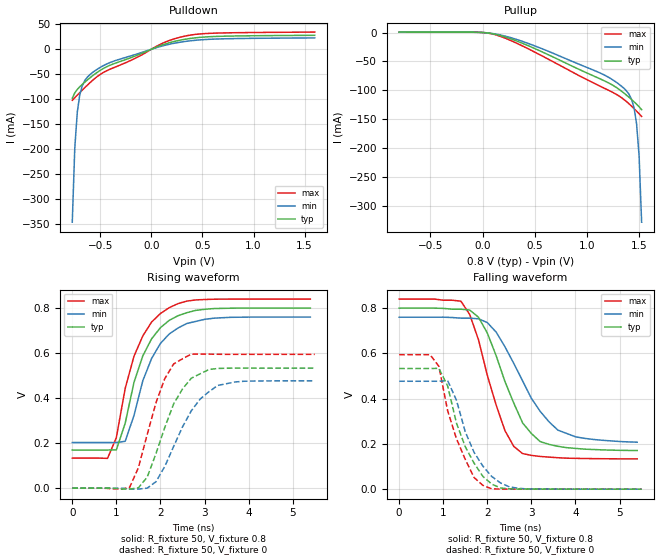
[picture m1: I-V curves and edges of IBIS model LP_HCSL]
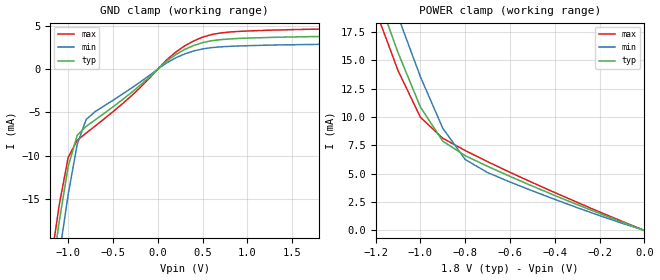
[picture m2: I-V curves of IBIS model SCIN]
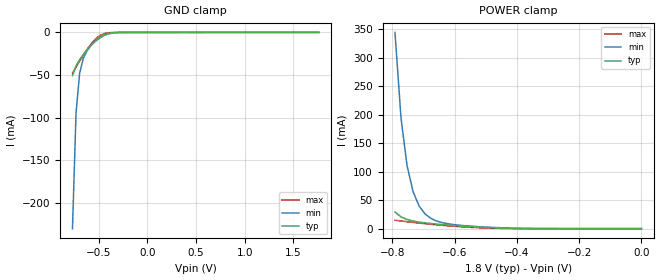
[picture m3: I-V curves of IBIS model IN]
| Integrated Devices Technolgy, Inc
[IBIS Ver]   4.1
[File name]   9dbu0431.ibs
[File Rev]   1.0
[Date]   Oct. 09, 2014
[Disclaimer] Integrated Device Technology, Inc. ("IDT") hereby grants the
   user of this ibis model a non-exclusive, nontransferable
   license to use this ibis model under the following terms. the
   user is granted this license only to use the ibis model and is
   not granted rights to sell, copy (except as needed to run the
   ibis model), rent, lease or sub-license the ibis model in
   whole or in part, or in modified form to anyone. the user may
   modify the ibis model to suit its specific applications, but
   rights to derivative works and such modifications shall belong
   to idt. this ibis model is provided on an as is" basis and idt
   makes absolutely no warranty with respect to the information
   contained herein. idt disclaims and customer waives all
   warranties, express and implied, including warranties of
   merchantability and fitness for a particular purpose. the
   entire risk as to quality and performance is with the user
   accordingly, in no event shall idt be liable for any direct or
   indirect damages, whether in contract or tort, including any
   lost profits or other incidental, consequential, exemplary, or
   punitive damages arising out of the use or application of the
   ibis model. further, idt reserves the right to make changes
   without notice to any product herein to improve reliability,
   function, or design. idt does not convey any license under
   patent rights or any other intellectual property rights,
   including those of third parties. idt is not obligated to
   provide maintenance or support for the licensed ibis model.
[Copyright]   Copyright 2012, Integrated Devices Technolgy, Inc. all rights
   reserved
[Component]   9dbu0431
[Manufacturer] Integrated Device Technology, Inc.
[Package]
|32-VFQFPN
|variable   typ   min   max
R_pkg   81.1m   62.2m   100.0m
L_pkg   6.7nH   4.9nH   8.5nH
C_pkg   0.53pF   0.21pF   0.85pF
[Pin] signal_name  model_name
1 ^vHIBW_BYPM_LOBW#   IN
2 FB_DNC   LP_HCSL
3 FB_DNC#   LP_HCSL
4 VDDR1.5   POWER
5 CLK_IN   CLKIN
6 CLK_IN#   CLKIN
7 GNDR   GND
8 GNDDIG   GND
9 VDDDIG1.5   POWER
10 SCLK_3.3   SCIN
11 SDATA_3.3   SCIN
12 vOE0#   IN
13 DIF0   LP_HCSL
14 DIF0#   LP_HCSL
15 GND   GND
16 VDDO1.5   POWER
17 vOE1#   IN
18 DIF1   LP_HCSL
19 DIF1#   LP_HCSL
20 GNDA   GND
21 VDDA1.5   POWER
22 DIF2   LP_HCSL
23 DIF2#   LP_HCSL
24 vOE2#   IN
25 VDDO1.5   POWER
26 GND   GND
27 DIF3   LP_HCSL
28 DIF3#   LP_HCSL
29 vOE3#   IN
30 GND   GND
31 ^CKPWRGD_PD#   PD
32 SADR_tri   IN
[Diff Pin]  inv_pin  vdiff tdelay_typ tdelay_min  tdelay_max
13   14   NA   0   0   0
17   18   NA   0   0   0
| Models and submodels in the file (5): LP_HCSL (Output), SCIN (Input), IN (Input), CLKIN (Input), PD (Input)
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[Model]   LP_HCSL
Model_type   Output
Polarity   Non-Inverting
|   typ   min   max
C_comp   2pF   1.5pF   2.5pF
Vmeas = 0.4V
Rref = 50
Cref = 0
Vref = 0.4V
|   typ   min   max
[Voltage range]   0.8V   0.76V   0.84V
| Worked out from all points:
|   slope of the pulldown table from 0 to 0.12 V, typ, clamps not added: 12.6 ohm
|   slope of the pullup table from 0 to 0.12 V, typ, clamps not added: 40.4 ohm
|   rising waveform, R_fixture 50, V_fixture 0.8: 20-80 % time 633ps typ, 641ps min, 627ps max; typ from 0.169 V to 0.8 V
|   falling waveform, R_fixture 50, V_fixture 0.8: 20-80 % time 760ps typ, 973ps min, 640ps max; typ from 0.8 V to 0.171 V
|   rising waveform, R_fixture 50, V_fixture 0: 20-80 % time 648ps typ, 750ps min, 540ps max; typ from 0 V to 0.533 V
|   falling waveform, R_fixture 50, V_fixture 0: 20-80 % time 591ps typ, 611ps min, 563ps max; typ from 0.533 V to 0 V
[Pulldown]
|Voltage   I (typ)   I (min)   I (max)
|Note, modeling breaks down at 250mA and above.  This is well beyond the functional   |
|operating range of the device.  Should this scenario occur, catastrophic failure and   |
|possible damage to the device and/or board is of higher concern than the I-V curve   |
|behavior.  The IBIS checker will flag currents in excess of 10A with warnings.  Lines   |
|with currents in excess of 0.35 A have been commented out.  The points still remain|
|available to the user if the user desires to use them.   |
|-8.00000e-01   -1.18956e-01   -6.48321e-01   -1.07624e-01
-775.5mV  -98.23mA   -346.4mA   -102.3mA
-751mV    -87.43mA   -198mA     -97.14mA
-726.5mV  -80.52mA   -126.3mA   -92.02mA
-702mV    -75.15mA   -91.19mA   -86.94mA
-677.6mV  -70.41mA   -73.06mA   -81.92mA
-628.6mV  -61.7mA    -56.11mA   -72.13mA
-579.6mV  -53.61mA   -47.04mA   -62.91mA
-359.2mV  -28.39mA   -23.18mA   -36.07mA
106.1mV   8.578mA    6.556mA    11.68mA
326.5mV   19.84mA    15.45mA    26.21mA
620.4mV   25.5mA     20.31mA    32.18mA
1.6V      27.87mA    22.65mA    34.32mA
[Pullup]
|Voltage   I (typ)   I (min)   I (max)
|Note, modeling breaks down at 250mA and above.  This is well beyond the functional   |
|operating range of the device.  Should this scenario occur, catastrophic failure and   |
|possible damage to the device and/or board is of higher concern than the I-V curve   |
|behavior.  The IBIS checker will flag currents in excess of 10A with warnings.  Lines   |
|with currents in excess of 0.35 A have been commented out.  The points still remain|
|available to the user if the user desires to use them.   |
-800mV    720.8uA    674uA      687.8uA
-48.48mV  366.7uA    329uA      361.2uA
121.2mV   -3.014mA   -2.451mA   -3.786mA
606.1mV   -36.3mA    -30.55mA   -43.69mA
1.139V    -80.99mA   -70.87mA   -93.7mA
1.309V    -98.03mA   -89.24mA   -109.6mA
1.406V    -112mA     -106.7mA   -123.2mA
1.43V     -115.8mA   -115.3mA   -127.2mA
1.455V    -119.8mA   -130mA     -131.5mA
1.479V    -123.9mA   -157.7mA   -135.9mA
1.503V    -128.3mA   -213.4mA   -140.4mA
1.527V    -133.4mA   -327.8mA   -145mA
| 1.55152e+00   -1.40006e-01   -5.61449e-01   -1.49713e-01
| 1.57576e+00   -1.50454e-01   -1.02014e+00   -1.54462e-01
| 1.60000e+00   -1.70613e-01   -1.84947e+00   -1.59268e-01
[Ramp]
|   typ   min   max
dV/dt_r   0.322/0.652n   0.288/0.756n   0.359/0.544n
dV/dt_f   0.377/0.759n   0.331/0.973n   0.423/0.64n
R_load =   50
[Rising Waveform]
R_fixture = 50
V_fixture = 0.8   |Vcc_typ
V_fixture_min = 0.76 |Vcc_min
V_fixture_max = 0.84 |Vcc_max
C_fixture = 0.0p
| Time   typ   min   max
0s        169.4mV    202.7mV    133.6mV
800ps     169.4mV    202.7mV    132.5mV
1ns       170.3mV    202.6mV    224.9mV
1.2ns     288.2mV    208.4mV    442.8mV
1.4ns     470.3mV    322.9mV    586.2mV
1.6ns     587.8mV    477.4mV    676.4mV
2ns       713mV      643mV      775.9mV
2.4ns     766.1mV    711.6mV    819.8mV
3ns       794.4mV    749.8mV    837.9mV
5.4ns     800mV      760mV      840mV
[Falling Waveform]
R_fixture = 50
V_fixture = 0.8   |Vcc_typ
V_fixture_min = 0.76 |Vcc_min
V_fixture_max = 0.84 |Vcc_max
C_fixture = 0.0p
| Time   typ   min   max
0s        800mV      760mV      840mV
1.4ns     795.4mV    755.9mV    830.8mV
1.6ns     791.6mV    755.7mV    772.3mV
1.8ns     759.8mV    753mV      660mV
2ns       689.9mV    736.2mV    503mV
2.4ns     475.8mV    629.3mV    258.6mV
2.8ns     292.8mV    478.6mV    157.3mV
3.2ns     210.1mV    343.6mV    144.6mV
3.6ns     189.4mV    261mV      139mV
5.4ns     170.7mV    207.6mV    133.8mV
[Rising Waveform]
R_fixture = 50
V_fixture = 0
C_fixture = 0.0p
| Time   typ   min   max
0s        36.65nV    422.2nV    16.59nV
1.3ns     -4.214mV   -3.249mV   3.128mV
1.5ns     1.766mV    -4.053mV   90.98mV
1.7ns     49.12mV    109.5uV    238.7mV
1.9ns     154.6mV    29.05mV    380.5mV
2.1ns     270.8mV    97.03mV    487.3mV
2.5ns     440.5mV    272.2mV    574.7mV
2.9ns     507.8mV    395.6mV    595.4mV
3.3ns     531.7mV    456.3mV    594.8mV
5.5ns     533mV      476.8mV    594.4mV
[Falling Waveform]
R_fixture = 50
V_fixture = 0
C_fixture = 0.0p
| Time   typ   min   max
0s        533mV      476.9mV    594.4mV
700ps     533mV      476.9mV    594.2mV
900ps     534.1mV    476.8mV    543.6mV
1.1ns     456.1mV    479.9mV    346.4mV
1.3ns     292mV      393mV      223.1mV
1.5ns     187.5mV    253.1mV    131.6mV
1.9ns     56.28mV    101.6mV    16.79mV
2.3ns     5.253mV    27.26mV    387.4uV
2.7ns     410.2uV    4.104mV    300.6uV
5.5ns     22.66uV    49.02uV    7.861uV
|   Model SCIN
[Model]   SCIN
Model_type   Input
Vinl =   0.54V
Vinh =   1.26V
C_comp   3.40pF   2.85pF   3.95pF
[Temperature Range]   25.00   70.00   0.000
[Voltage Range]   1.80V   1.62V   1.98V
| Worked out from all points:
|   GND clamp passes 1 mA (typ) near -0.10 V on its own axis
|   POWER clamp passes 1 mA (typ) near -0.13 V on its own axis
[GND_clamp]
| voltage   I(typ)   I(min)   I(max)
-1.8V     -72.89mA   -76.87mA   -70.76mA
-1.2V     -24.92mA   -29.01mA   -22.79mA
-1.1V     -17.6mA    -21.48mA   -15.68mA
-1V       -11.25mA   -14.47mA   -10.2mA
-900mV    -7.66mA    -8.72mA    -8.23mA
-800mV    -6.62mA    -5.82mA    -7.39mA
-300mV    -2.76mA    -2.24mA    -3.14mA
100mV     920uA      720uA      1.08mA
300mV     2.27mA     1.75mA     2.68mA
600mV     3.28mA     2.48mA     3.99mA
900mV     3.54mA     2.67mA     4.35mA
1.8V      3.76mA     2.86mA     4.62mA
[POWER_clamp]
| voltage   I(typ)   I(min)   I(max)
-1.8V     57.31mA    60.73mA    55.47mA
-1.2V     21.16mA    24.54mA    19.4mA
-1.1V     15.67mA    18.87mA    14.09mA
-1V       10.87mA    13.54mA    9.97mA
-900mV    7.86mA     9mA        8.12mA
-800mV    6.59mA     6.25mA     7.04mA
-700mV    5.65mA     5.1mA      6.06mA
-600mV    4.76mA     4.27mA     5.12mA
-300mV    2.28mA     2.01mA     2.48mA
0V        44.83pA    370pA      23.45pA
|   Model IN
[Model]   IN
Model_type   Input
Polarity   Non-Inverting
Vinl = 0.63V
Vinh = 1.17V
|   typ   min   max
C_comp   2pF   1.5pF   2.5pF
|   typ   min   max
[Voltage range]   1.8V   1.7V   1.9V
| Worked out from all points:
|   GND clamp passes 1 mA (typ) near -0.39 V on its own axis
|   POWER clamp passes 1 mA (typ) near -0.45 V on its own axis
[GND_clamp]
|Voltage   I (typ)   I (min)   I (max)
|Note, modeling breaks down at 250mA and above.  This is well beyond the functional   |
|operating range of the device.  Should this scenario occur, catastrophic failure and   |
|possible damage to the device and/or board is of higher concern than the I-V curve   |
|behavior.  The IBIS checker will flag currents in excess of 10A with warnings.  Lines   |
|with currents in excess of 0.35 A have been commented out.  The points still remain|
|available to the user if the user desires to use them.   |
|-1.80000e+00   -4.43726e+01   -4.17458e+01   -4.86820e+01
|-1.76327e+00   -4.25922e+01   -4.02056e+01   -4.65395e+01
|-1.72653e+00   -4.08117e+01   -3.86654e+01   -4.43969e+01
|-1.68980e+00   -3.90312e+01   -3.71251e+01   -4.22544e+01
|-1.65306e+00   -3.72507e+01   -3.55849e+01   -4.01118e+01
|-1.61633e+00   -3.54702e+01   -3.40446e+01   -3.79693e+01
|-1.57959e+00   -3.36896e+01   -3.25043e+01   -3.58267e+01
|-1.54286e+00   -3.19091e+01   -3.09640e+01   -3.36840e+01
|-1.50612e+00   -3.01285e+01   -2.94236e+01   -3.15414e+01
|-1.46939e+00   -2.83479e+01   -2.78833e+01   -2.93987e+01
|-1.43265e+00   -2.65672e+01   -2.63429e+01   -2.72561e+01
|-1.39592e+00   -2.47866e+01   -2.48025e+01   -2.51134e+01
|-1.35918e+00   -2.30059e+01   -2.32621e+01   -2.29707e+01
|-1.32245e+00   -2.12253e+01   -2.17217e+01   -2.08279e+01
|-1.28571e+00   -1.94446e+01   -2.01813e+01   -1.86852e+01
|-1.24898e+00   -1.76639e+01   -1.86409e+01   -1.65424e+01
|-1.21224e+00   -1.58832e+01   -1.71005e+01   -1.43996e+01
|-1.17551e+00   -1.41025e+01   -1.55600e+01   -1.22568e+01
|-1.13878e+00   -1.23218e+01   -1.40196e+01   -1.01141e+01
|-1.10204e+00   -1.05411e+01   -1.24792e+01   -7.97124e+00
|-1.06531e+00   -8.76046e+00   -1.09388e+01   -5.82843e+00
|-1.02857e+00   -6.97978e+00   -9.39848e+00   -3.68562e+00
|-9.91837e-01   -5.19912e+00   -7.85813e+00   -1.54785e+00
|-9.55102e-01   -3.41847e+00   -6.31781e+00   -3.90595e-01
|-9.18367e-01   -1.63807e+00   -4.77753e+00   -1.29996e-01
|-8.81633e-01   -5.21907e-01   -3.23728e+00   -7.87800e-02
|-8.44898e-01   -1.73459e-01   -1.69709e+00   -6.40873e-02
|-8.08163e-01   -7.85613e-02   -6.33127e-01   -5.54276e-02
-771.4mV  -50.63mA   -230.2mA   -47.85mA
-734.7mV  -39.27mA   -94.07mA   -40.58mA
-698mV    -32.06mA   -48.05mA   -33.55mA
-661.2mV  -26.07mA   -30.55mA   -26.83mA
-624.5mV  -20.62mA   -22.01mA   -20.51mA
-587.8mV  -15.64mA   -16.46mA   -14.75mA
-514.3mV  -7.457mA   -8.514mA   -5.771mA
-477.6mV  -4.509mA   -5.592mA   -2.97mA
-404.1mV  -1.167mA   -1.846mA   -517.4uA
-293.9mV  -74.63uA   -181.5uA   -23.43uA
1.763V    14.13uA    10.16uA    21.47uA
[Power_clamp]
|Voltage   I (typ)   I (min)   I (max)
|Note, modeling breaks down at 250mA and above.  This is well beyond the functional   |
|operating range of the device.  Should this scenario occur, catastrophic failure and   |
|possible damage to the device and/or board is of higher concern than the I-V curve   |
|behavior.  The IBIS checker will flag currents in excess of 10A with warnings.  Lines   |
|with currents in excess of 0.35 A have been commented out.  The points still remain|
|available to the user if the user desires to use them.   |
|-1.80000e+00   5.60662e+01   5.31750e+01   6.07752e+01
|-1.78061e+00   5.48637e+01   5.21252e+01   5.93477e+01
|-1.76122e+00   5.36611e+01   5.10754e+01   5.79201e+01
|-1.74184e+00   5.24586e+01   5.00255e+01   5.64925e+01
|-1.72245e+00   5.12561e+01   4.89757e+01   5.50649e+01
|-1.70306e+00   5.00535e+01   4.79259e+01   5.36374e+01
|-1.68367e+00   4.88510e+01   4.68761e+01   5.22098e+01
|-1.66429e+00   4.76485e+01   4.58263e+01   5.07822e+01
|-1.64490e+00   4.64460e+01   4.47765e+01   4.93547e+01
|-1.62551e+00   4.52434e+01   4.37267e+01   4.79271e+01
|-1.60612e+00   4.40409e+01   4.26769e+01   4.64996e+01
|-1.58673e+00   4.28384e+01   4.16272e+01   4.50720e+01
|-1.56735e+00   4.16359e+01   4.05774e+01   4.36444e+01
|-1.54796e+00   4.04334e+01   3.95276e+01   4.22169e+01
|-1.52857e+00   3.92308e+01   3.84778e+01   4.07893e+01
|-1.50918e+00   3.80283e+01   3.74280e+01   3.93618e+01
|-1.48980e+00   3.68258e+01   3.63783e+01   3.79342e+01
|-1.47041e+00   3.56233e+01   3.53285e+01   3.65067e+01
|-1.45102e+00   3.44208e+01   3.42787e+01   3.50791e+01
|-1.43163e+00   3.32183e+01   3.32290e+01   3.36516e+01
|-1.41224e+00   3.20159e+01   3.21792e+01   3.22241e+01
|-1.39286e+00   3.08134e+01   3.11294e+01   3.07965e+01
|-1.37347e+00   2.96109e+01   3.00797e+01   2.93690e+01
|-1.35408e+00   2.84084e+01   2.90300e+01   2.79415e+01
|-1.33469e+00   2.72059e+01   2.79802e+01   2.65140e+01
|-1.31531e+00   2.60035e+01   2.69305e+01   2.50865e+01
|-1.29592e+00   2.48010e+01   2.58808e+01   2.36589e+01
|-1.27653e+00   2.35986e+01   2.48310e+01   2.22314e+01
|-1.25714e+00   2.23961e+01   2.37813e+01   2.08039e+01
|-1.23776e+00   2.11937e+01   2.27316e+01   1.93764e+01
|-1.21837e+00   1.99912e+01   2.16819e+01   1.79490e+01
|-1.19898e+00   1.87888e+01   2.06322e+01   1.65215e+01
|-1.17959e+00   1.75864e+01   1.95825e+01   1.50940e+01
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-791.8mV  29.26mA    344.8mA    14.84mA
-772.4mV  20.73mA    194.3mA    13.49mA
-753.1mV  16.1mA     110.7mA    12.21mA
-733.7mV  13.35mA    64.84mA    10.99mA
-714.3mV  11.49mA    39.63mA    9.831mA
-694.9mV  10.08mA    25.65mA    8.721mA
-675.5mV  8.904mA    17.72mA    7.666mA
-636.7mV  6.907mA    10.16mA    5.729mA
-539.8mV  3.07mA     4.093mA    2.051mA
-365.3mV  167.9uA    383.5uA    57.09uA
0V        14.13nA    10.08nA    21.48nA
